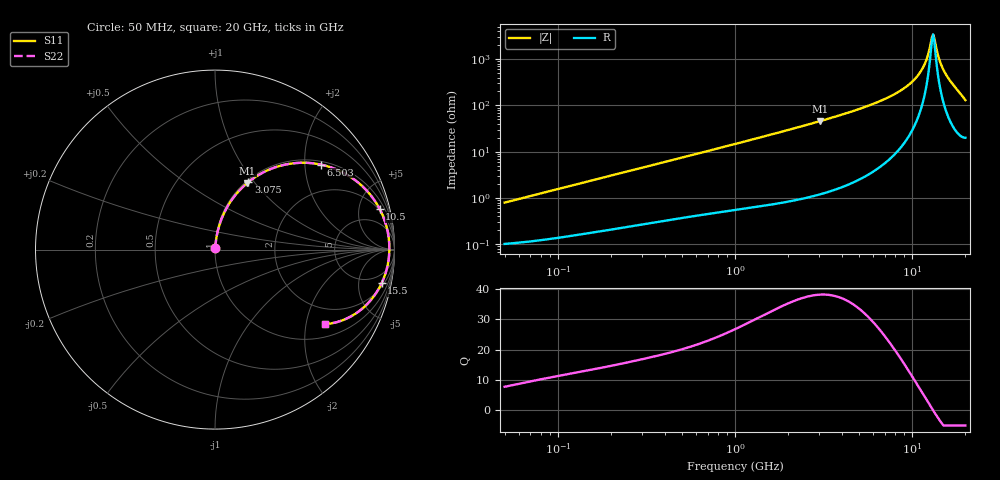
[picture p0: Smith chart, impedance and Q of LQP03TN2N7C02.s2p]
!Murata Part Number: LQP03TN2N7C02
!These Parameters are Measured in Series Mode Connection
!  o--[Z]--o
!Port1  Port2
!  o-------o
!Freq. Start=50[MHz] Stop=20[GHz], 401[Steps]
# Hz S RI R 50
!Freq.(Hz) S11(Real) S11(Imag) S21(Real) S21(Imag) S12(Real) S12(Imag) S22(Real) S22(Imag)
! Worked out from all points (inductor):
!   401 points, 50 MHz to 20 GHz, reference 50 ohm
!   read as one part in series: L = 2.51 nH near 51.52 MHz
!   highest Q = 38.1 at 3.03 GHz (marker M1), where L = 2.41 nH
!   self-resonance near 12.95 GHz
!   S11 on the Smith chart (normalised r, x): 50 MHz: 1.00, +0.02; 3.075 GHz: 1.02, +0.93; 6.503 GHz: 1.09, +2.43; 10.5 GHz: 1.85, +7.81; 15.5 GHz: 2.56, -9.32; 20 GHz: 1.40, -2.57
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5e7  0.00108 0.00789  0.9989 -0.00789  0.9989 -0.00789  0.00108 0.00789
1.364002e8  0.00209 0.021  0.9979 -0.021  0.9979 -0.021  0.00209 0.021
3.721004e8  0.00614 0.0552  0.9939 -0.0552  0.9939 -0.0552  0.00614 0.0552
1e9  0.0262 0.1421  0.9738 -0.1421  0.9738 -0.1421  0.0262 0.1421
1.766834e9  0.0696 0.2401  0.9304 -0.2401  0.9304 -0.2401  0.0696 0.2401
2.728004e9  0.1502 0.3443  0.8498 -0.3443  0.8498 -0.3443  0.1502 0.3443
3.029571e9  0.1804 0.3717  0.8196 -0.3717  0.8196 -0.3717  0.1804 0.3717
3.075291e9  0.1852 0.3756  0.8148 -0.3756  0.8148 -0.3756  0.1852 0.3756
4.472136e9  0.3461 0.4619  0.6539 -0.4619  0.6539 -0.4619  0.3461 0.4619
6.503449e9  0.5923 0.4731  0.4077 -0.4731  0.4077 -0.4731  0.5923 0.4731
7.442007e9  0.6937 0.4392  0.3063 -0.4392  0.3063 -0.4392  0.6937 0.4392
9.041845e9  0.8329 0.3417  0.1671 -0.3417  0.1671 -0.3417  0.8329 0.3417
1.050288e10  0.9176 0.226  0.0824 -0.226  0.0824 -0.226  0.9176 0.226
1.166392e10  0.9561 0.1265  0.0439 -0.1265  0.0439 -0.1265  0.9561 0.1265
1.220001e10  0.9658 0.0801  0.0342 -0.0801  0.0342 -0.0801  0.9658 0.0801
1.276073e10  0.9709 0.0319  0.0291 -0.0319  0.0291 -0.0319  0.9709 0.0319
1.314879e10  0.9715 -0.000992  0.0285 0.000992  0.0285 0.000992  0.9715 -0.000992
1.354865e10  0.9697 -0.0344  0.0303 0.0344  0.0303 0.0344  0.9697 -0.0344
1.438523e10  0.9585 -0.1022  0.0415 0.1022  0.0415 0.1022  0.9585 -0.1022
1.550395e10  0.9285 -0.1873  0.0715 0.1873  0.0715 0.1873  0.9285 -0.1873
1.747767e10  0.8339 -0.3171  0.1661 0.3171  0.1661 0.3171  0.8339 -0.3171
2e10  0.612 -0.4156  0.388 0.4156  0.388 0.4156  0.612 -0.4156
